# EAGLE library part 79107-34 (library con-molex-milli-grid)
RECEPTACAL
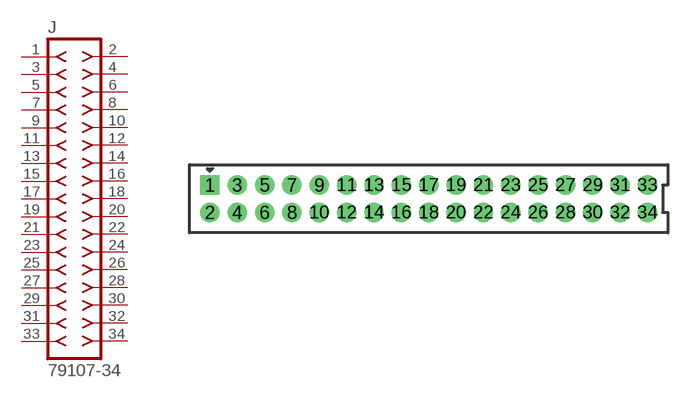
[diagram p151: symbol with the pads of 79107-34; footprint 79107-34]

Designator prefix J

## 79107-34  [79107-34]
1  1  pas
2  2  pas
3  3  pas
4  4  pas
5  5  pas
6  6  pas
7  7  pas
8  8  pas
9  9  pas
10  10  pas
11  11  pas
12  12  pas
13  13  pas
14  14  pas
15  15  pas
16  16  pas
17  17  pas
18  18  pas
19  19  pas
20  20  pas
21  21  pas
22  22  pas
23  23  pas
24  24  pas
25  25  pas
26  26  pas
27  27  pas
28  28  pas
29  29  pas
30  30  pas
31  31  pas
32  32  pas
33  33  pas
34  34  pas

## Footprint 79107-34 (pad centres in mm)
RECEPTACAL Dual Row, Vertical, Through-Hole
drill 0.914 square: 1 -16,1
drill 0.914: 2 -16,-1; 3 -14,1; 4 -14,-1; 5 -12,1; 6 -12,-1; 7 -10,1; 8 -10,-1; 9 -8,1; 10 -8,-1; 11 -6,1; 12 -6,-1; 13 -4,1; 14 -4,-1; 15 -2,1; 16 -2,-1; 17 0,1; 18 0,-1; 19 2,1; 20 2,-1; 21 4,1; 22 4,-1; 23 6,1; 24 6,-1; 25 8,1; 26 8,-1; 27 10,1; 28 10,-1; 29 12,1; 30 12,-1; 31 14,1; 32 14,-1; 33 16,1; 34 16,-1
